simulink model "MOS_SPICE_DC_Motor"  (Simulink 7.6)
settings: Solver=ode15s  StartTime=0.0  StopTime=12  RelTol=1e-3
StopFcn:
  | close all, clc
  | load pos_vit.mat
  | plot(x(1,:),x(2,:), x(1,:),x(3,:))
  | grid
  | title('Vitesse et Position angulaires')
  | xlabel('temps')
  | 
  | figure
  | load Ve_Idrain.mat
  | plotyy(y(1,:),y(2,:), y(1,:),y(3,:))
  | grid
  | title('Tension de commande et Courant drain du MOS')
  | xlabel('temps')
libraries: fl_lib x10, elec_lib x7, nesl_utility x5

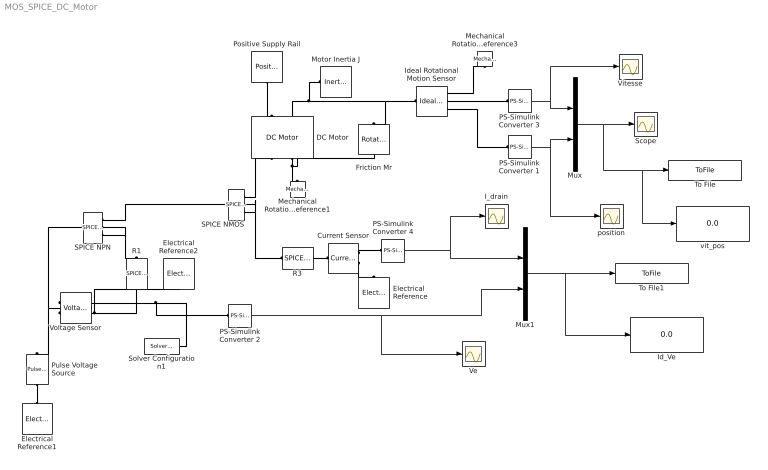
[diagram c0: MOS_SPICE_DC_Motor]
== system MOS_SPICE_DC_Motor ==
  Current Sensor : fl_lib/Electrical/Electrical Sensors/Current Sensor  DialogController=NetworkEngine.DynNeDlgSource  SystemSampleTime=-1  i1_Log=off  v1_Log=off  LocalVarNames=|i1|v1  LocalVarDescs=|i1|v1  LocalVarLogging=[0 0]
  DC Motor : elec_lib/Actuators & Drivers/Rotational Actuators/DC Motor  DialogController=NetworkEngine.DynNeDlgSource  SystemSampleTime=-1  parameterization=1  Ra=3.9 Ohm  La=1.2e-05 H  emf_or_torque=1  Kv=7.2e-05 V/rpm  Ki=6.876e-04 N*m/A  T_stall=2.4e-04 N*m  w_max=1.91e+04 rpm  w_rated=1.5e+04 rpm  P_rated=0.08 W  V_rated=1.5 V  J=0.01 g*cm^2  lam=1e-08 N*m/(rad/s)  speed0=0 rpm  current_Log=off  voltage_Log=off  power_Log=off  i2r_Log=off  torque_Log=off  speed_Log=off  LocalVarNames=|current|voltage|power|i2r|torque|speed  LocalVarDescs=|Current (A)|Voltage (V)|Power (W)|Electrical losses (W)|Torque (Nm)|Angular speed (rad/s)  LocalVarLogging=[0 0 0 0 0 0]
  Electrical Reference : fl_lib/Electrical/Electrical Elements/Electrical Reference  DialogController=NetworkEngine.DynNeDlgSource  SystemSampleTime=-1  i_Log=off  LocalVarNames=|i  LocalVarDescs=|i  LocalVarLogging=0
  Electrical Reference1 : fl_lib/Electrical/Electrical Elements/Electrical Reference  DialogController=NetworkEngine.DynNeDlgSource  SystemSampleTime=-1  i_Log=off  LocalVarNames=|i  LocalVarDescs=|i  LocalVarLogging=0
  Electrical Reference2 : fl_lib/Electrical/Electrical Elements/Electrical Reference  DialogController=NetworkEngine.DynNeDlgSource  SystemSampleTime=-1  i_Log=off  LocalVarNames=|i  LocalVarDescs=|i  LocalVarLogging=0
  Friction Mr : fl_lib/Mechanical/Rotational Elements/Rotational Friction  DialogController=NetworkEngine.DynNeDlgSource  SystemSampleTime=-1  brkwy_trq=1e-6 N*m  Col_trq=1e-6 N*m  visc_coef=0 N*m/(rad/s)  trans_coef=10 s/rad  vel_thr=0.1 rad/s  t_Log=off  w_Log=off  LocalVarNames=|friction_torque|rel_velocity|power  LocalVarDescs=|Friction torque (N*m)|Relative velocity (rad/s)|Power (W)  LocalVarLogging=[0 0 0]
  I_drain : Scope
  Id_Ve : Display
  Ideal Rotational Motion Sensor : fl_lib/Mechanical/Mechanical Sensors/Ideal Rotational Motion Sensor  DialogController=NetworkEngine.DynNeDlgSource  SystemSampleTime=-1  offset=0 rad  w_Log=off  t_Log=off  phi_Log=off  LocalVarNames=|w|t|phi  LocalVarDescs=|w|t|phi  LocalVarLogging=[0 0 0]
  Mechanical Rotational Reference1 : fl_lib/Mechanical/Rotational Elements/Mechanical Rotational Reference  DialogController=NetworkEngine.DynNeDlgSource  SystemSampleTime=-1  t_Log=off  LocalVarNames=|t  LocalVarDescs=|t  LocalVarLogging=[]
  Mechanical Rotational Reference3 : fl_lib/Mechanical/Rotational Elements/Mechanical Rotational Reference  DialogController=NetworkEngine.DynNeDlgSource  SystemSampleTime=-1  t_Log=off  LocalVarNames=|t  LocalVarDescs=|t  LocalVarLogging=[]
  Motor Inertia J : fl_lib/Mechanical/Rotational Elements/Inertia  DialogController=NetworkEngine.DynNeDlgSource  SystemSampleTime=-1  inertia=10 g*cm^2  initial_velocity=0 rad/s  t_Log=off  LocalVarNames=|torque|velocity  LocalVarDescs=|Inertia torque (N*m)|Inertia absolute velocity (rad/s)  LocalVarLogging=[0 0]
  Mux : Mux  Inputs=2
  Mux1 : Mux  Inputs=2
  PS-Simulink Converter {1..4} (4 alike) : nesl_utility/PS-Simulink Converter  DialogController=NetworkEngine.DynNeUtilDlgSource  SystemSampleTime=-1  PhysicalDomain=network_engine_domain  LeftPortType=input  RightPortType=output  SubClassName=ps_output  Unit=1  AffineConversion=off
  Positive Supply Rail : elec_lib/Sources/Positive Supply Rail  DialogController=NetworkEngine.DynNeDlgSource  SystemSampleTime=-1  v0=24 V  current_Log=off  voltage_Log=off  power_Log=off  LocalVarNames=|current|voltage|power  LocalVarDescs=|Current (A)|Voltage (V)|Power (W)  LocalVarLogging=[0 0 0]
  Pulse Voltage  Source : elec_lib/Additional Components/SPICE-Compatible Components/Sources/Pulse Voltage Source  DialogController=NetworkEngine.DynNeDlgSource  SystemSampleTime=-1  V1=0 V  V2=12 V  TD=1 s  TR=0.2 s  TF=1e-9 s  PW=5 s  PER=Inf s  voltage_Log=off  LocalVarNames=|voltage  LocalVarDescs=|Voltage (V)  LocalVarLogging=0
  R1 : elec_lib/Additional Components/SPICE-Compatible Components/Passive Devices/SPICE Resistor  DialogController=NetworkEngine.DynNeDlgSource  SystemSampleTime=-1  SCALE=1  R_param=1  R=100 Ohm  RSH=0 Ohm  LENGTH=1e-6 m  WIDTH=1e-6 m  NARROW=0 m  T_param=1  TC1=0 1/K  TC2=0 1/K^2  TOFFSET=0 K  TFIXED=300.15 K  TMEAS=300.15 K  LocalVarLogging=[]
  R3 : elec_lib/Additional Components/SPICE-Compatible Components/Passive Devices/SPICE Resistor  DialogController=NetworkEngine.DynNeDlgSource  SystemSampleTime=-1  SCALE=1  R_param=1  R=0.1 Ohm  RSH=0 Ohm  LENGTH=1e-6 m  WIDTH=1e-6 m  NARROW=0 m  T_param=1  TC1=0 1/K  TC2=0 1/K^2  TOFFSET=0 K  TFIXED=300.15 K  TMEAS=300.15 K  LocalVarLogging=[]
  SPICE NMOS : elec_lib/Additional Components/SPICE-Compatible Components/Semiconductor Devices/SPICE NMOS  DialogController=NetworkEngine.DynNeDlgSource  SystemSampleTime=-1  AREA=1  SCALE=1  LENGTH=1e-4 m  WIDTH=1e-4 m  AD=0 m^2  AS=0 m^2  PD=0 m  PS=0 m  NRD=1  NRS=1  LEVEL=1  VTO=0 V  KP=2e-5 A/V^2  GAMMA=0 V^0.50000  PHI=0.6 V  LAMBDA=0 1/V  RD=0.01 Ohm  RS=1e-4 Ohm  C_param=1  CBD=0 F  CBS=0 F  IS=1e-14 A  ND=1  PB=0.8 V  CGSO=0 F/m  CGDO=0 F/m  CGBO=0 F/m  RSH=NaN Ohm  CJ=0 F/m^2  MJ=0.5  CJSW=0 F/m  MJSW=0.5  JS=0 A/m^2  TOX=NaN m  LD=0 m  U0=600 cm^2/s/V  FC=0.5  NSUB=NaN 1/cm^3  TPG=1  NSS=0 1/cm^2  UEXP=0  UCRIT=1e+4 V/cm  NEFF=1  DELTA=0  VMAX=0 m/s  XJ=0 m  NFS=0 1/cm^2  ETA=0  THETA=0 1/V  KAPPA=0.2  T_param=1  TOFFSET=0 K  TFIXED=300.15 K  TMEAS=300.15 K  IC_given=1  ICVDS=0 V  ICVGS=0 V  ICVBS=0 V  MTYPE=1  LocalVarLogging=[]
  SPICE NPN : elec_lib/Additional Components/SPICE-Compatible Components/Semiconductor Devices/SPICE NPN  DialogController=NetworkEngine.DynNeDlgSource  SystemSampleTime=-1  AREA=1 m^2  SCALE=1  IS=1e-16 A/m^2  BF=100  NF=1  VAF=Inf V  IKF=Inf A/m^2  ISE=0 A/m^2  NE=1.5  BR=1  NR=1  VAR=Inf V  IKR=Inf A/m^2  ISC=0 A/m^2  NC=2  RB=1 m^2*Ohm  IRB=Inf A/m^2  RBM=0 m^2*Ohm  RE=1e-4 m^2*Ohm  RC=0.01 m^2*Ohm  C_param=1  CJE=0 F/m^2  VJE=0.75 V  MJE=0.33  TF=0 s  XTF=0  VTF=Inf V  ITF=0 A/m^2  CJC=0 F/m^2  VJC=0.75 V  MJC=0.33  XCJC=1  TR=0 s  CJS=0 F/m^2  VJS=0.75 V  MJS=0  T_param=1  XTB=0  EG=1.11 eV  XTI=3  FC=0.5  TOFFSET=0 K  TFIXED=300.15 K  TMEAS=300.15 K  IC_given=1  ICVBE=0 V  ICVCE=0 V  LocalVarLogging=[]
  Scope : Scope
  Solver Configuration1 : nesl_utility/Solver Configuration  DialogController=NetworkEngine.DynNeUtilDlgSource  SystemSampleTime=-1  PhysicalDomain=network_engine_domain  LeftPortType=input  RightPortType=generic  SubClassName=solver  Accelerate=off  Profile=off  ResidualTolerance=1e-9  MaxNonlinIter=12  MaxModeIter=2  DoFixedCost=off  UseLocalSampling=off  DoDC=off  LinearAlgebra=Full  LocalSolverSampleTime=.001  LocalSolverChoice=NE_BACKWARD_EULER_ADVANCER  UseLocalSolver=off
  To File : ToFile  Filename=pos_vit.mat  MatrixName=x
  To File1 : ToFile  Filename=Ve_Idrain  MatrixName=y
  Ve : Scope
  Vitesse : Scope
  Voltage Sensor : fl_lib/Electrical/Electrical Sensors/Voltage Sensor  DialogController=NetworkEngine.DynNeDlgSource  SystemSampleTime=-1  i1_Log=off  v1_Log=off  LocalVarNames=|i1|v1  LocalVarDescs=|i1|v1  LocalVarLogging=[0 0]
  position : Scope
  vit_pos : Display
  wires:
  PS-Simulink Converter 3/1 -> Mux/1, Vitesse/1
  Mux/1 -> Scope/1, To File/1, vit_pos/1
  PS-Simulink Converter 1/1 -> Mux/2, position/1
  PS-Simulink Converter 2/1 -> Mux1/2, Ve/1
  PS-Simulink Converter 4/1 -> Mux1/1, I_drain/1
  Mux1/1 -> To File1/1, Id_Ve/1
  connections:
  SPICE NMOS/RConn1 -- DC Motor/RConn1
  SPICE NMOS/RConn3 -- SPICE NMOS/RConn2 -- R3/LConn1
  SPICE NPN/LConn1 -- Pulse Voltage  Source/LConn1 -- Voltage Sensor/LConn1
  Pulse Voltage  Source/RConn1 -- Electrical Reference1/LConn1
  DC Motor/RConn2 -- Mechanical Rotational Reference1/LConn1 -- Friction Mr/RConn1
  Ideal Rotational Motion Sensor/LConn1 -- DC Motor/LConn2 -- Motor Inertia J/LConn1 -- Friction Mr/LConn1
  Ideal Rotational Motion Sensor/RConn1 -- Mechanical Rotational Reference3/LConn1
  PS-Simulink Converter 3/LConn1 -- Ideal Rotational Motion Sensor/RConn2
  Ideal Rotational Motion Sensor/RConn3 -- PS-Simulink Converter 1/LConn1
  Current Sensor/RConn2 -- Electrical Reference/LConn1
  Voltage Sensor/RConn1 -- PS-Simulink Converter 2/LConn1 -- Solver Configuration1/RConn1
  Current Sensor/RConn1 -- PS-Simulink Converter 4/LConn1
  SPICE NPN/RConn2 -- R1/LConn1 -- SPICE NPN/RConn3
  Positive Supply Rail/RConn1 -- DC Motor/LConn1
  Voltage Sensor/RConn2 -- Electrical Reference2/LConn1 -- R1/RConn1
  R3/RConn1 -- Current Sensor/LConn1
  SPICE NMOS/LConn1 -- SPICE NPN/RConn1
